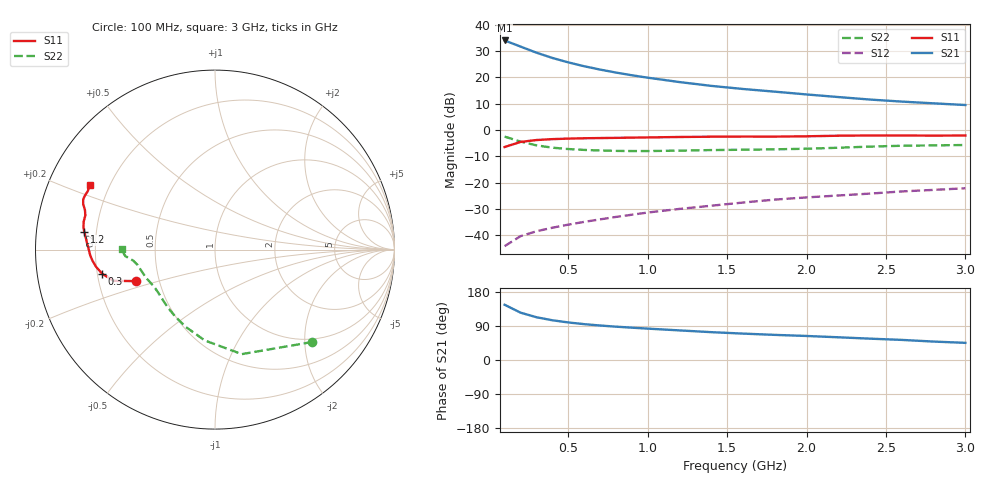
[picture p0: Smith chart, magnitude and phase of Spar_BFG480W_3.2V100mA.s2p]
! Filename: 3_2100BFG480.001
! Title: BFG480W
! Bias: Vce=3.2V; Ic=100mA
! Company: NXP Semiconductors NL
! User: Quality&Reliability T&D
! Measure time: 10 Nov 1999 / 11:57:59
#  MHz  S  MA  R 50
! Freq  S11  S21  S12  S22  :
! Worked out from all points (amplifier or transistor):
!   20 points, 100 MHz to 3 GHz, reference 50 ohm
!   highest |S21| = 34.1 dB at 100 MHz (marker M1)
!   |S21| within 3 dB of that: start of sweep to 229.2 MHz
!   unconditionally stable (mu >= 1): 685 MHz to end of sweep
!   at 400 MHz: K = 0.83, MSG = 32.3 dB, |S12| = -37.2 dB
!   at 1.2 GHz: K = 1.08, MAG = 22.4 dB, |S12| = -30.1 dB
!   at 3 GHz: K = 1.06, MAG = 14.4 dB, |S12| = -22.2 dB
!   S11 on the Smith chart (normalised r, x): 100 MHz: 0.37, -0.17; 300 MHz: 0.22, -0.10; 1.2 GHz: 0.15, +0.06; 3 GHz: 0.13, +0.24
100  0.4729 -158.2  50.44 145.8  0.006149 69.1  0.7473 -43.5
200  0.5914 -162.9  38.61 125.0  0.009521 61.0  0.6013 -75.6
300  0.6427 -167.9  29.55 112.9  0.0118 60.1  0.5094 -96.4
400  0.669 -171.7  23.46 104.9  0.01378 61.9  0.4605 -110.7
500  0.6843 -174.6  19.33 99.1  0.01578 63.9  0.4334 -120.9
600  0.6952 -177.1  16.31 94.6  0.01781 65.7  0.4172 -128.5
700  0.701 -179.2  14.1 91.1  0.01987 67.9  0.4066 -134.3
800  0.7071 178.8  12.37 88.0  0.02213 69.6  0.3998 -139.2
900  0.7145 177.0  10.99 85.3  0.02435 71.2  0.3968 -143.4
1000  0.7204 175.3  9.882 82.8  0.02684 72.2  0.3968 -147.1
1200  0.7346 172.4  8.154 78.1  0.03144 73.6  0.4042 -153.0
1400  0.7439 170.2  6.899 73.5  0.03619 74.4  0.4141 -157.4
1600  0.7482 167.8  6.019 69.7  0.04155 75.1  0.4204 -160.8
1800  0.7471 165.2  5.353 66.3  0.04732 75.5  0.4278 -164.4
2000  0.7574 163.1  4.738 63.4  0.05205 76.1  0.4395 -168.7
2200  0.7765 161.0  4.227 60.0  0.05661 75.9  0.4587 -172.2
2400  0.7855 159.2  3.787 56.3  0.06154 75.4  0.4824 -174.4
2600  0.7851 157.6  3.463 53.0  0.06765 74.6  0.5006 -175.8
2800  0.78 155.3  3.209 48.6  0.0724 73.2  0.5092 -177.6
3000  0.7847 152.6  2.98 45.2  0.07774 72.4  0.5167 179.5
